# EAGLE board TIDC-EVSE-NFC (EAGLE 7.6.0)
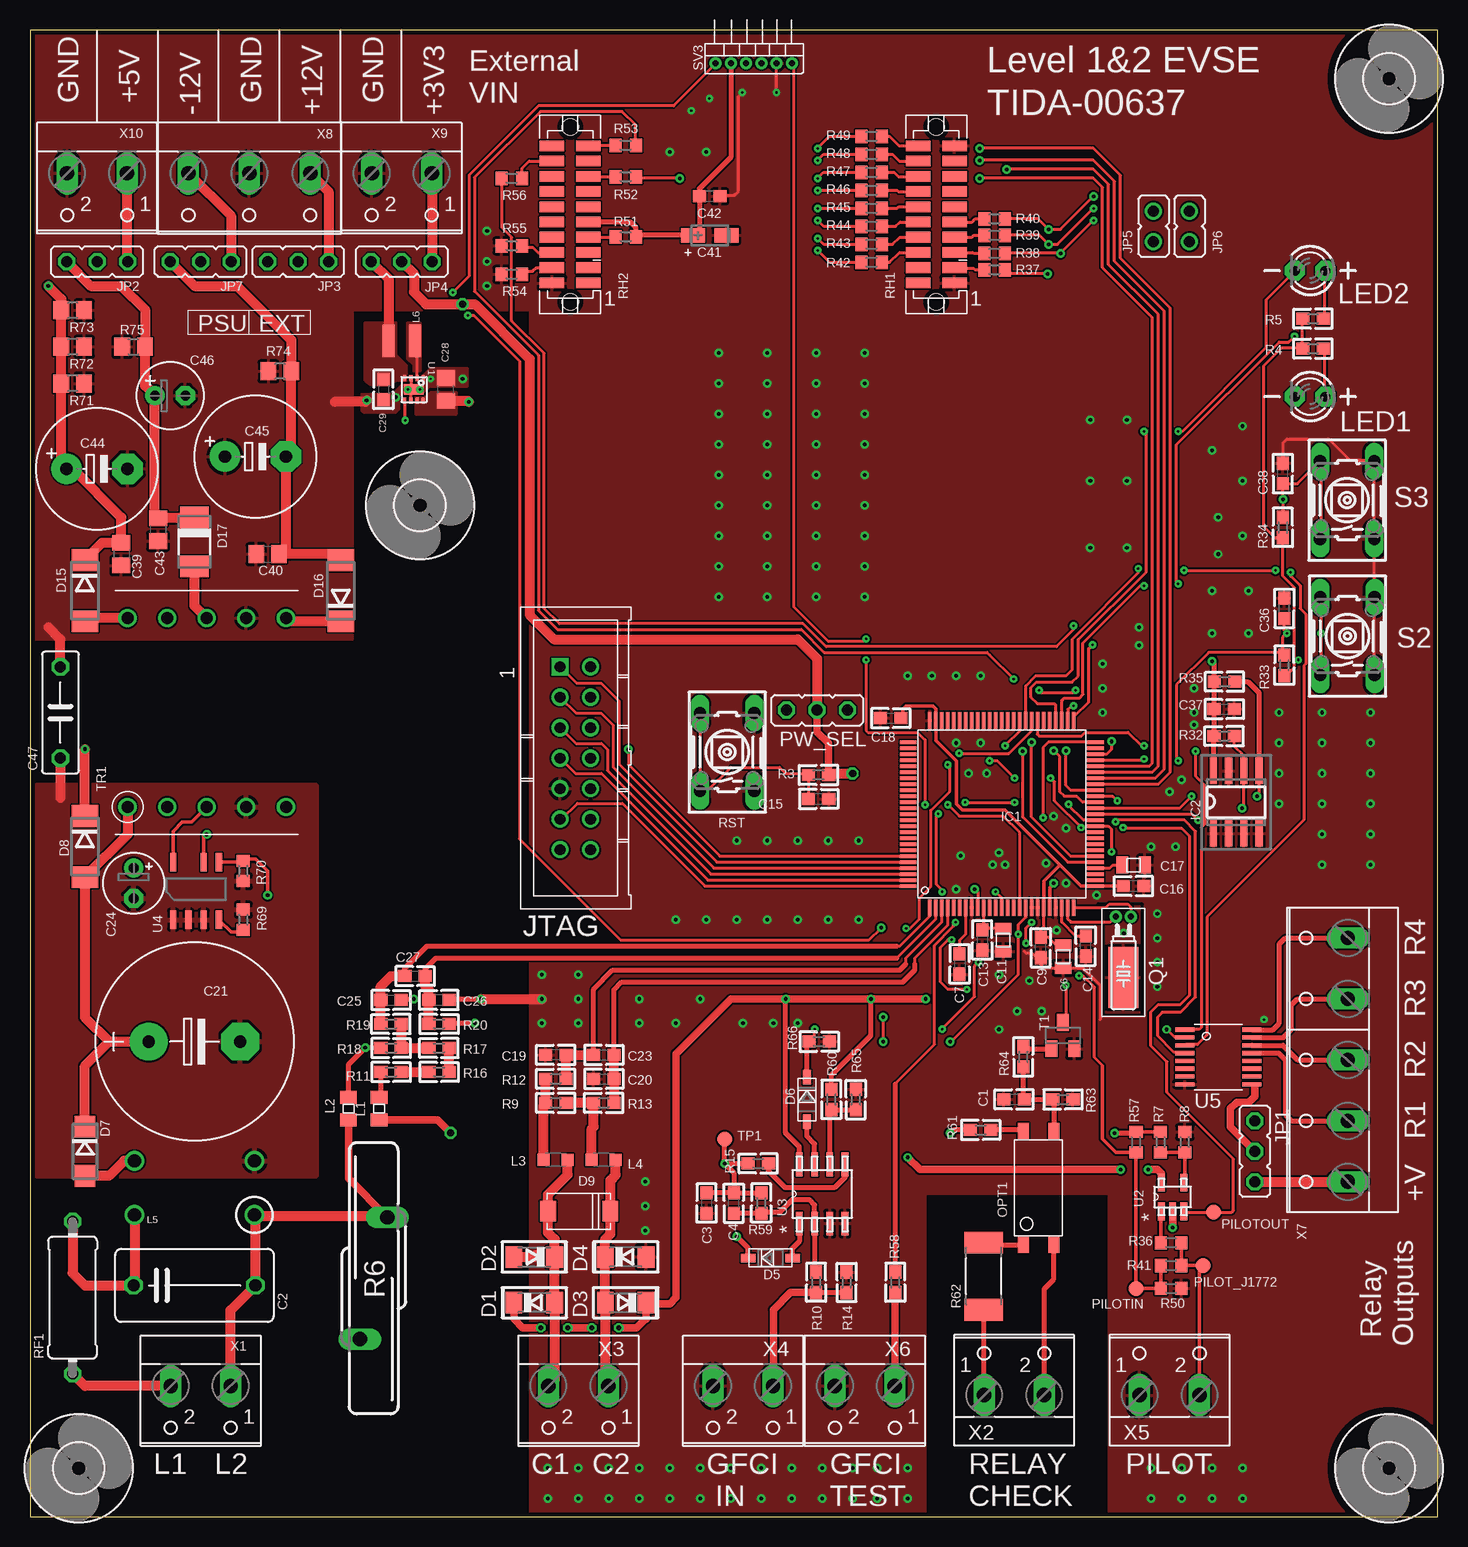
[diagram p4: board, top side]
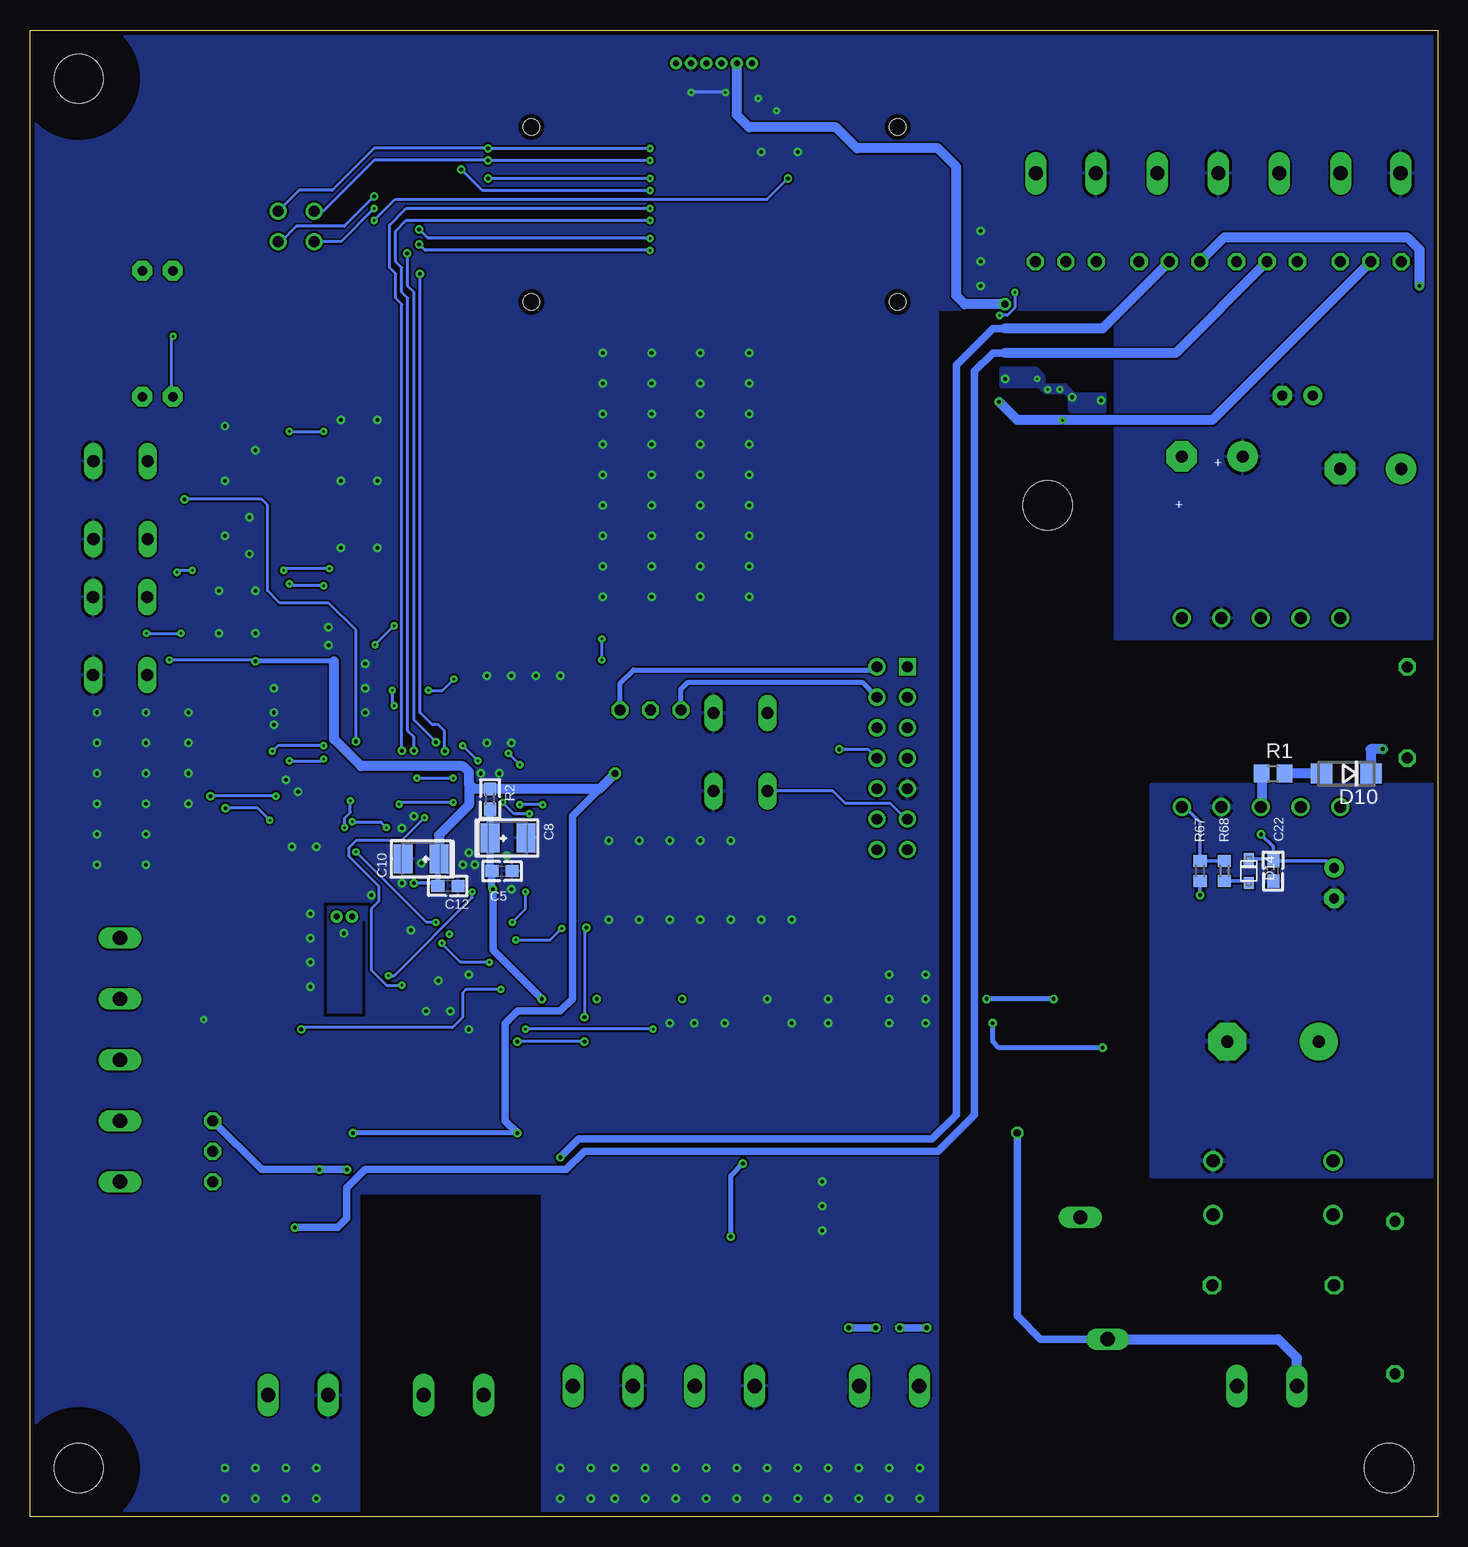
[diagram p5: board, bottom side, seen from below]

Size 117.35 x 123.95 mm. Coordinates in mm from the lower left corner, seen from the top.
Outline: 117.35,0 117.35,123.95 0,123.95 0,0 117.35,0
Copper layers (1*16): Top 0.0356mm / dielectric 1.5011mm / Bottom 0.0356mm
Design rules "typical_4pcb *": minimum track width 10mil, minimum drill 8mil, track to track 6mil, track to pad 6mil, pad to pad 6mil, via to via 6mil, smd to smd 6mil, copper to edge 15mil, drill to drill 8mil, minimum pad ring 10mil, minimum via ring 8mil, stop-mask expansion 4mil, vias tented up to drill 25mil, thermal gap 10mil
tRestrict: 4 lines
bRestrict: 4 lines

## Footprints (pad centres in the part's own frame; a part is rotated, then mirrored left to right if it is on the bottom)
C0603 = smd 1.1 x 1: 1 -0.85,0; 2 0.85,0
C102-064X133 = drill 1.016 octagon: 1 -5.08,0; 2 5.08,0
0805 = smd 1 x 1.4: 1 -0.94,0; 2 0.94,0
SMC_B = smd 1.6 x 2.4: + -1.5,0; - 1.5,0
E7,5-16 = drill 1.016 pad 3.15: + -3.81,0 | drill 1.016 pad 3.15 octagon: - 3.81,0
E2,5-5 = drill 0.813 pad 1.6: + -1.27,0 | drill 0.813 pad 1.6 octagon: - 1.27,0
C0805 = smd 1.3 x 1.5: 1 -0.95,0; 2 0.95,0
CT3216 = smd 2 x 1.2: + -1.4,0; - 1.4,0
E5-10,5 = drill 1.016 pad 2.54: + -2.54,0 | drill 1.016 pad 2.54 octagon: - 2.54,0
E2,5-6 = drill 0.813 pad 1.6: + -1.27,0 | drill 0.813 pad 1.6 octagon: - 1.27,0
C075-032X103 = drill 0.914 octagon: 1 -3.81,0; 2 3.81,0
SOD80C = smd 1.4 x 1.8: A -1.7,0; C 1.7,0
SOD-123 = smd 1.2 x 0.7: A 1.85,0; C -1.85,0
DO214AC = smd 1.8 x 1.7: A 2.05,0; C -2.05,0
DO214AA = smd 1.8 x 2.2: A 2.55,0; C -2.55,0
DO-214 = smd 1.3 x 1.7: 1 0,0; 2 5.2,0
SOD-323F = smd 1 x 0.8: A -1,0; C 1,0
DO-214AC = smd 1.8 x 2.4: A 2.025,0; C -2.025,0
4,1 = hole 4.1: 0,0
PZ100 = smd 1.4 x 0.3: 1 -7.8,6; 2 -7.8,5.5; 3 -7.8,5; 4 -7.8,4.5; 5 -7.8,4; 6 -7.8,3.5; 7 -7.8,3; 8 -7.8,2.5; 9 -7.8,2; 10 -7.8,1.5; 11 -7.8,1; 12 -7.8,0.5; 13 -7.8,0; 14 -7.8,-0.5; 15 -7.8,-1; 16 -7.8,-1.5; 17 -7.8,-2; 18 -7.8,-2.5; 19 -7.8,-3; 20 -7.8,-3.5; 21 -7.8,-4; 22 -7.8,-4.5; 23 -7.8,-5; 24 -7.8,-5.5; 25 -7.8,-6; 51 7.8,-6; 52 7.8,-5.5; 53 7.8,-5; 54 7.8,-4.5; 55 7.8,-4; 56 7.8,-3.5; 57 7.8,-3; 58 7.8,-2.5; 59 7.8,-2; 60 7.8,-1.5; 61 7.8,-1; 62 7.8,-0.5; 63 7.8,0; 64 7.8,0.5; 65 7.8,1; 66 7.8,1.5; 67 7.8,2; 68 7.8,2.5; 69 7.8,3; 70 7.8,3.5; 71 7.8,4; 72 7.8,4.5; 73 7.8,5; 74 7.8,5.5; 75 7.8,6 | smd 0.3 x 1.4: 26 -6,-7.8; 27 -5.5,-7.8; 28 -5,-7.8; 29 -4.5,-7.8; 30 -4,-7.8; 31 -3.5,-7.8; 32 -3,-7.8; 33 -2.5,-7.8; 34 -2,-7.8; 35 -1.5,-7.8; 36 -1,-7.8; 37 -0.5,-7.8; 38 0,-7.8; 39 0.5,-7.8; 40 1,-7.8; 41 1.5,-7.8; 42 2,-7.8; 43 2.5,-7.8; 44 3,-7.8; 45 3.5,-7.8; 46 4,-7.8; 47 4.5,-7.8; 48 5,-7.8; 49 5.5,-7.8; 50 6,-7.8; 76 6,7.8; 77 5.5,7.8; 78 5,7.8; 79 4.5,7.8; 80 4,7.8; 81 3.5,7.8; 82 3,7.8; 83 2.5,7.8; 84 2,7.8; 85 1.5,7.8; 86 1,7.8; 87 0.5,7.8; 88 0,7.8; 89 -0.5,7.8; 90 -1,7.8; 91 -1.5,7.8; 92 -2,7.8; 93 -2.5,7.8; 94 -3,7.8; 95 -3.5,7.8; 96 -4,7.8; 97 -4.5,7.8; 98 -5,7.8; 99 -5.5,7.8; 100 -6,7.8
SO-08 = smd 2.2 x 0.6: 1 -2.6,1.905; 2 -2.6,0.635; 3 -2.6,-0.635; 4 -2.6,-1.905; 5 2.6,-1.905; 6 2.6,-0.635; 7 2.6,0.635; 8 2.6,1.905
JP2 = drill 0.914 octagon: 1 -2.54,0; 2 0,0; 3 2.54,0
JP1 = drill 0.914: 1 0,-1.27; 2 0,1.27
MA07-2JTAG = drill 0.9 pad 1.422 square: 1 0,0 | drill 0.9 pad 1.422: 2 0,2.54; 3 2.54,0; 4 2.54,2.54; 5 5.08,0; 6 5.08,2.54; 7 7.62,0; 8 7.62,2.54; 9 10.16,0; 10 10.16,2.54; 11 12.7,0; 12 12.7,2.54; 13 15.24,0; 14 15.24,2.54
0805@1 = smd 1.092 x 1.397: 1 -0.94,0; 2 0.94,0
L2012C = smd 1 x 1: 1 -1,0; 2 1,0
744821110 = drill 1.1: 1 5,-2.25; 2 5,2.25; 3 -5,2.25; 4 -5,-2.25
SRN3015 = smd 2.7 x 1: V_1 0,1.1; V_2 0,-1.1
LED3MM = drill 0.8 pad 1.676 octagon: A -1.27,0; K 1.27,0
TCLT1600 = smd 1.3 x 0.9: 1 -4.75,1.27; 2 -4.75,-1.27; 3 4.75,-1.27; 4 4.75,1.27
B1,27 = smd 1.27 x 1.27: TP 0,0
TC26H-1 = drill 0.5 pad 1.016: 1 -0.635,0; 2 0.635,0 | smd 2.54 x 5.08: 3 0,5.08
R0805 = smd 1.3 x 1.5: 1 -0.95,0; 2 0.95,0
R0603 = smd 1.1 x 1: 1 -0.85,0; 2 0.85,0
S20K680-1 = drill 1.2 long: 1 -1.143,-5.08; 2 1.143,5.08
R0603' = smd 1 x 1.1: 1 -0.85,0; 2 0.85,0
R2512 = smd 1.8 x 3.2: 1 -2.8,0; 2 2.8,0
0411/12 = drill 0.914 octagon: 1 -6.35,0; 2 6.35,0
TFM-110-02-SM-D-A-K = smd 2.032 x 0.889: 1 -1.524,5.715; 2 1.524,5.715; 3 -1.524,4.445; 4 1.524,4.445; 5 -1.524,3.175; 6 1.524,3.175; 7 -1.524,1.905; 8 1.524,1.905; 9 -1.524,0.635; 10 1.524,0.635; 11 -1.524,-0.635; 12 1.524,-0.635; 13 -1.524,-1.905; 14 1.524,-1.905; 15 -1.524,-3.175; 16 1.524,-3.175; 17 -1.524,-4.445; 18 1.524,-4.445; 19 -1.524,-5.715; 20 1.524,-5.715 | hole 1.359: 0,7.303; 0,-7.303
B3F-10XX = drill 1.016 long: 1 -3.251,2.261; 2 3.251,2.261; 3 -3.251,-2.261; 4 3.251,-2.261
MA06-1-1.27 = drill 0.5 pad 0.9: 1 0,0; 2 1.27,0; 3 2.54,0; 4 3.81,0; 5 5.08,0; 6 6.35,0
SOT23 = smd 1 x 1.4: 1 -0.95,-1.1; 2 0.95,-1.1; 3 0,1.1
RLTI-1118 = drill 1: V_1 -7.874,6.604; V_2 -7.874,3.302; V_3 -7.874,0; V_4 -7.874,-3.302; V_5 -7.874,-6.604; V_6 7.874,-6.604; V_7 7.874,-3.302; V_8 7.874,0; V_9 7.874,3.302; V_10 7.874,6.604
DSG0008A = smd 0.508 x 0.254: 1 -0.94,0.762; 2 -0.94,0.254; 3 -0.94,-0.254; 4 -0.94,-0.762; 5 0.94,-0.762; 6 0.94,-0.254; 7 0.94,0.254; 8 0.94,0.762 | smd 0.889 x 1.6: 9 0,0
DBV5 = smd 1.473 x 0.559: 1 -1.194,0.94; 2 -1.194,0; 3 -1.194,-0.94; 4 1.194,-0.94; 5 1.194,0.94
M08A = smd 1.981 x 0.559: 1 -2.464,1.905; 2 -2.464,0.635; 3 -2.464,-0.635; 4 -2.464,-1.905; 5 2.464,-1.905; 6 2.464,-0.635; 7 2.464,0.635; 8 2.464,1.905
D0007A = smd 1.524 x 0.508: 1 0,3.81; 2 0,2.54; 3 0,1.27; 4 0,0; 5 4.801,0; 6 4.801,1.27; 8 4.801,3.81
TSSOP_16 = smd 1.6 x 0.35: V_1 -2.8,4.55; V_2 -2.8,3.9; V_3 -2.8,3.25; V_4 -2.8,2.6; V_5 -2.8,1.95; V_6 -2.8,1.3; V_7 -2.8,0.65; V_8 -2.8,0; V_9 2.8,0; V_10 2.8,0.65; V_11 2.8,1.3; V_12 2.8,1.95; V_13 2.8,2.6; V_14 2.8,3.25; V_15 2.8,3.9; V_16 2.8,4.55
W237-102 = drill 1.194 long: 1 -2.5,-1.27; 2 2.5,-1.27
W237-5P = drill 1.194 long: 1 -10.16,-0.635; 2 -5.08,-0.635; 3 0,-0.635; 4 5.08,-0.635; 5 10.16,-0.635
W237-133 = drill 1.194 long: 1 -5.08,-0.635; 2 0,-0.635; 3 5.08,-0.635

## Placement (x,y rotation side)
C1  47pF  [C0603]  82.04,34.8 180 top
C2  [C102-064X133]  13.72,19.3 0 top
C3  10u  [C0603]  56.39,26.16 270 top
C4  100n  [C0603]  58.67,26.16 90 top
C5  0.1uF  [C0603]  78,53.84 0 bottom
C6  4.7uF  [0805]  86.12,46.71 90 top
C7  0.1uF  [C0603]  77.5,46.09 270 top
C8  4.7uF  [SMC_B]  77.5,56.59 0 bottom
C9  4.7uF  [C0603]  84.25,47.46 90 top
C10  4.7uF  [SMC_B]  84.75,54.84 180 bottom
C11  4.7uF  [0805]  81.12,48.09 90 top
C12  0.1uF  [C0603]  82.5,52.59 180 bottom
C13  0.1uF  [C0603]  79.38,48.09 270 top
C14  0.47uF  [C0603]  88,47.59 90 top
C15  0.01uF  [C0603]  65.74,59.86 0 top
C16  0.47uF  [C0603]  92,52.59 180 top
C17  4.7uF  [0805]  92,54.34 180 top
C18  0.1uF  [C0603]  71.75,66.59 0 top
C19  47pF  [C0603]  43.83,38.52 180 top
C20  47pF  [C0603]  47.83,36.52 0 top
C21  [E7,5-16]  13.72,39.62 0 top
C22  .1u  [C0603]  13.72,53.85 90 bottom
C23  15nF  [C0603]  47.83,38.52 0 top
C24  22u  [E2,5-5]  8.64,52.83 270 top
C25  47pF  [C0603]  30.1,43.09 0 top
C26  47pF  [C0603]  34.1,43.09 180 top
C27  15nF  [C0603]  32.1,45.09 0 top
C28  4.7u  [C0805]  34.67,93.98 90 top
C29  10.0u  [C0603]  29.46,93.98 270 top
C36  0.1uF  [C0603]  104.56,75.74 90 top
C37  0.1uF  [C0603]  99.56,67.34 0 top
C38  0.1uF  [C0603]  104.44,86.98 90 top
C39  1u  [C0805]  7.62,80.26 270 top
C40  1u  [C0805]  19.81,80.26 0 top
C41  10uF  [CT3216]  56.66,106.83 0 top
C42  0.1uF  [C0603]  56.66,110.08 180 top
C43  1u  [C0805]  10.67,82.3 270 top
C44  680u  [E5-10,5]  5.59,87.38 0 top
C45  680u  [E5-10,5]  18.8,88.39 0 top
C46  220u  [E2,5-6]  11.68,93.47 0 top
C47  1000p  [C075-032X103]  2.54,67.06 90 top
D1  1N4148  [SOD80C]  42.04,17.87 180 top
D2  1N4148  [SOD80C]  42.04,21.68 0 top
D3  1N4148  [SOD80C]  49.66,17.87 0 top
D4  1N4148  [SOD80C]  49.66,21.68 180 top
D5  [SOD-123]  61.72,21.59 0 top
D6  [SOD-123]  64.77,34.8 270 top
D7  [DO214AC]  4.57,30.48 270 top
D8  [DO214AA]  4.57,55.88 270 top
D9  SMAJ5.0CA  [DO-214]  48.39,25.49 180 top
D10  [DO214AC]  7.62,61.98 180 bottom
D14  [SOD-323F]  15.75,53.85 90 bottom
D15  [DO214AA]  4.57,77.22 270 top
D16  [DO214AA]  25.91,77.22 90 top
D17  [DO-214AC]  13.72,81.28 270 top
H1  MOUNT-HOLE4.1  [4,1]  4.06,4.06 0 top
H2  MOUNT-HOLE4.1  [4,1]  113.28,4.06 0 top
H3  MOUNT-HOLE4.1  [4,1]  113.28,119.89 0 top
H4  MOUNT-HOLE4.1  [4,1]  32.51,84.33 0 top
IC1  F6733---PZ100  [PZ100]  81,58.59 90 top
IC2  24C02CSN  [SO-08]  100.56,59.59 90 top
JP1  [JP2]  102.11,30.48 270 top
JP2  [JP2]  5.59,104.65 180 top
JP3  [JP2]  22.35,104.65 180 top
JP4  [JP2]  30.99,104.65 180 top
JP5  [JP1]  93.66,107.58 0 top
JP6  [JP1]  96.66,107.58 0 top
JP7  [JP2]  14.22,104.65 180 top
JTAG  [MA07-2JTAG]  44.2,70.87 270 top
L1  EXCML20A  [0805@1]  29.09,34.04 90 top
L2  EXCML20A  [0805@1]  26.54,34.04 90 top
L3  BLM21BD121SN1D  [L2012C]  43.83,29.77 180 top
L4  BLM21BD121SN1D  [L2012C]  47.83,29.77 180 top
L5  744821110  [744821110]  13.72,27.43 0 top
L6  1u  [SRN3015]  30.99,98.04 90 top
LED1  [LED3MM]  106.71,93.38 180 top
LED2  [LED3MM]  106.71,103.88 180 top
OPT1  TCLT1600  [TCLT1600]  84.07,27.43 90 top
PILOT_J1772  TPB1,27  [B1,27]  97.79,20.95 270 top
PILOTIN  TPB1,27  [B1,27]  92.2,19.05 90 top
PILOTOUT  TPB1,27  [B1,27]  98.68,25.4 270 top
PW_SEL  [JP2]  65.62,67.26 180 top
Q1  32.768  [TC26H-1]  91.15,50.04 180 top
R1  33.2  [R0805]  13.72,61.98 0 bottom
R2  10 ohm  [R0603]  79,59.84 270 bottom
R3  47K  [R0603]  65.74,61.85 180 top
R4  100  [R0603]  106.96,97.38 180 top
R5  100  [R0603]  106.96,99.88 180 top
R6  S20K275  [S20K680-1]  28.65,19.89 180 top
R7  100k  [R0603']  94.23,31.24 90 top
R8  100k  [R0603']  96.27,31.24 270 top
R9  13R  [R0603]  43.83,34.52 180 top
R10  1K  [R0603]  65.53,19.56 270 top
R11  330K  [R0603]  30.1,37.09 0 top
R12  1K  [R0603]  43.83,36.52 180 top
R13  1K  [R0603]  47.83,34.52 180 top
R14  330  [R0603]  68.07,19.56 90 top
R15  150  [R0603]  60.71,29.46 180 top
R16  330K  [R0603]  34.1,37.09 0 top
R17  330K  [R0603]  34.1,39.09 180 top
R18  3K  [R0603]  30.1,39.09 0 top
R19  100  [R0603]  30.1,41.09 180 top
R20  1K  [R0603]  34.1,41.09 0 top
R32  10K  [R0603]  99.56,65.09 180 top
R33  100k  [R0603]  104.56,70.99 270 top
R34  100k  [R0603]  104.44,82.48 270 top
R35  10K  [R0603]  99.58,69.63 180 top
R36  910  [R0603']  95.12,22.86 0 top
R37  0  [R0603']  80.41,103.95 180 top
R38  0  [R0603']  80.41,105.33 180 top
R39  0  [R0603']  80.41,106.83 180 top
R40  0  [R0603']  80.41,108.2 180 top
R41  300k  [R0603']  95.12,20.95 0 top
R42  0  [R0603']  70.16,104.58 180 top
R43  0  [R0603']  70.16,106.08 180 top
R44  0  [R0603']  70.16,107.58 180 top
R45  0  [R0603']  70.16,109.08 180 top
R46  0  [R0603']  70.16,110.58 180 top
R47  0  [R0603']  70.16,112.08 180 top
R48  0  [R0603']  70.16,113.58 180 top
R49  0  [R0603']  70.16,115.08 180 top
R50  100k  [R0603']  95.12,19.05 180 top
R51  0  [R0603']  49.66,106.71 180 top
R52  0  [R0603']  49.66,111.71 180 top
R53  0  [R0603']  49.66,114.33 180 top
R54  0  [R0603']  40.16,103.58 180 top
R55  0  [R0603']  40.16,105.96 180 top
R56  0  [R0603']  40.16,111.58 180 top
R57  82k  [R0603']  92.2,31.24 90 top
R58  330  [R0603]  72.14,19.56 270 top
R59  100k  [R0603]  60.96,26.16 270 top
R60  150  [R0603]  66.8,34.8 270 top
R61  1K  [R0603]  79.25,32.26 0 top
R62  18k  [R2512]  79.5,20.07 90 top
R63  1K  [R0603]  86.11,34.8 0 top
R64  1K  [R0603]  82.8,38.35 90 top
R65  150  [R0603]  68.83,34.8 90 top
R66  10k  [R0603]  65.79,39.62 0 top
R67  33.2k  [R0603']  19.81,53.85 90 bottom
R68  10  [R0603']  17.78,53.85 90 bottom
R69  806  [R0603']  17.78,49.78 270 top
R70  15.0k  [R0603']  17.78,53.85 90 top
R71  2k  [R0805]  3.56,94.49 180 top
R72  2k  [R0805]  3.56,97.54 180 top
R73  2k  [R0805]  3.56,100.58 180 top
R74  2k  [R0805]  20.83,95.5 180 top
R75  511  [R0805]  8.64,97.54 0 top
RF1  [0411/12]  3.56,18.29 90 top
RH1  [TFM-110-02-SM-D-A-K]  75.55,108.58 180 top
RH2  [TFM-110-02-SM-D-A-K]  45.03,108.58 180 top
RST  [B3F-10XX]  58.12,63.76 90 top
S2  [B3F-10XX]  109.83,73.42 90 top
S3  [B3F-10XX]  109.8,84.76 90 top
SV3  [MA06-1-1.27]  57.16,121.19 0 top
T1  BC846  [SOT23]  86.11,40.13 0 top
TP1  TPB1,27  [B1,27]  57.91,31.5 90 top
TR1  RLTI-1118RLTI-1118  [RLTI-1118]  14.73,67.06 90 top
U1  TPS62063DSGR  [DSG0008A]  32,93.98 270 top
U2  OPA171  [DBV5]  95.25,26.67 90 top
U3  LM7321  [M08A]  66.04,26.92 90 top
U4  Value  [D0007A]  15.75,49.78 90 top
U5  TPL7407L  [TSSOP_16]  99.06,36.07 0 top
X1  [W237-102]  14.22,9.65 180 top
X2  [W237-102]  82.04,11.43 0 top
X3  [W237-102]  45.72,9.65 180 top
X4  [W237-102]  59.44,9.65 180 top
X5  [W237-102]  95,11.43 0 top
X6  [W237-102]  69.6,9.65 180 top
X7  [W237-5P]  109.22,38.1 90 top
X8  [W237-133]  18.29,111.38 180 top
X9  [W237-102]  30.99,110.74 180 top
X10  [W237-102]  5.59,110.74 180 top

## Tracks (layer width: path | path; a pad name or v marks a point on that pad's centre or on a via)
+3V3_S
  Top 0.813: JP4.3 29.89,103.21 L6.V_1
  pour Top (no thermals): 30.48,99.57 30.48,96.9 31.37,96.01 31.37,94.74 30.48,94.74 29.97,94.36 28.45,94.36 27.94,94.74 27.94,99.57
+5V  (via drill 0.2, 0.3)
  Top 0.254: v31.27,91.41 31.27,92.9 U1.5
  Top 0.813: v36.58,92.96 36.51,93.03 C28.1
  Bottom 0.254: v31.27,91.41 31.27,91.44
  Bottom 0.813: JP2.2 18.8,91.44 31.27,91.44 35.05,91.44 v36.58,92.96
  pour Top (no thermals): 35.56,93.73 33.4,93.73 33.02,93.34 32.13,93.34 32.13,91.95 35.56,91.95
+5V_S
  Top 0.813: D17.C 13.66,83.25 C43.1 10.41,83.5 C46.+ 9.59,94.3 R75.2 9.59,100.65 7.62,102.62 5.08,102.62 JP2.3
+12V  (via drill 0.3)
  Top 0.61: v73.15,29.97 74.17,28.96 v90.93,28.96 | v93.22,28.96 93.98,28.96 94.31,28.63 U2.5
  Bottom 0.61: v73.15,29.97 71.63,31.5 42.16,31.5 40.13,33.53 40.13,96.01 37.08,99.06 36.07,99.06 | JP1.1 98.04,28.96 v93.22,28.96 v90.93,28.96
  Bottom 0.813: JP3.2 27.94,99.06 36.07,99.06
+12V_S  (via drill 0.3)
  Top 0.813: D15.C 6.02,81.21 C39.1 7.62,83.31 3.56,87.38 C44.+ 2.61,87.82 R71.2 R72.2 R73.2 2.61,101.53 v1.52,102.62
  Bottom 0.813: JP3.3 17.78,106.68 2.54,106.68 1.52,105.66 v1.52,102.62
-12V  (via drill 0.3)
  Top 0.61: v95.25,24.13 U2.2
  Bottom 0.61: 36.07,97.03 37.08,97.03 38.61,95.5 38.61,33.53 41.66,30.48 71.12,30.48 72.64,28.96 89.41,28.96 90.93,27.43 90.93,24.89 91.69,24.13 v95.25,24.13
  Bottom 0.813: JP7.2 21.84,97.03 36.07,97.03
-12V_S
  Top 0.813: D16.A 25.41,80.26 C40.2 21.34,80.84 C45.- 21.78,88.83 R74.1 21.78,98.11 17.27,102.62 13.72,102.62 JP7.3
AVCC  (via drill 0.3, 0.38)
  Top 0.254: IC1.9 79,52.09 v78.75,52.34
  Top 0.406: R60.1 66.8,36.83 70.1,40.13 v70.1,43.18 | U3.8 64.14,30.86 62.99,32 v62.99,43.18
  Top 0.61: D1.C 40.34,16.51 41.08,15.77 v42.58,15.77 | v44.83,15.77 v46.83,15.77 | v49.08,15.77 50.58,15.77 51.36,16.54 D3.C | D3.C 51.36,16.49 | D3.C 51.44,17.78 53.34,17.78 53.85,18.29 53.85,38.61 58.42,43.18 v62.99,43.18 v70.1,43.18 v74.68,43.18
  Bottom 0.406: C5.1 79,54.24 | v78.75,52.34 78.85,52.44
  Bottom 0.61: R2.2 C8.+ 79,54.24 | 78.85,52.44 C5.1 | v78.75,52.34 | v42.58,15.77 v44.83,15.77 | v46.83,15.77 v49.08,15.77 | v74.68,43.18 78.75,47.25 v78.75,52.34
BT1  (via drill 0.3)
  Top 0.254: R34.1 104.46,83.5 v104.46,84.84 104.46,86.04 C38.1 105.66,86.13 S3.2 107.63,87.95 107.63,81.6 S3.1 | IC1.48 89.75,63.59 90.17,64.01 v90.17,64.64
  Bottom 0.254: v90.17,64.64 90.17,73.91 92.46,76.2 96.52,76.2 97.54,77.22 97.54,84.33 98.04,84.84 v104.46,84.84
BT2  (via drill 0.2)
  Top 0.254: 104.46,74.61 C36.1 | S2.2 107.63,76.52 v107.63,73.66 107.63,70.48 S2.1 | 104.78,74.61 C36.1 | v95.73,63.02 95.57,63.18 95.57,69.37 98.27,72.07 104.46,72.07 | 104.46,72.07 R33.1 | IC1.47 92.77,63.09 v92.87,63.18 | 104.46,72.07 104.46,73.34 v104.78,73.66 104.56,73.87 C36.1
  Top 0.406: C36.1 104.65,74.68
  Bottom 0.254: v107.63,73.66 v104.78,73.66 | v92.87,63.18 93.03,63.02 v95.73,63.02
CUR1+
  Top 0.813: L3.1 44.83,28.52 43.19,26.87 D9.2 43.19,23.7 43.74,23.15 D2.C D1.A 43.74,11.44 X3.2
CUR1-
  Top 0.813: L4.1 48.83,28.52 48.39,28.07 D9.1 48.39,23.58 47.96,23.15 D4.C D3.A 47.96,11.19 X3.1
DVCC  (via drill 0.2, 0.3, 0.6)
  Top 0.254: 98.65,62.1 IC2.8 | 106.05,97.47 106.05,99.69 R5.2 | 105.41,71.44 105.41,70.8 104.78,70.17 R33.2 | 105.41,71.44 105.41,77.47 104.46,78.42 104.46,81.6 R34.2 104.14,81.6 103.82,81.6 102.87,82.55 102.87,95.99 104.35,97.47 106.05,97.47 | 106.05,97.47 R4.2 | v105.73,71.44 105.41,71.44
  Top 0.305: R7.2 R57.2 | IC1.21 85,52.49 v85.34,52.83
  Top 0.406: IC2.8 98.65,65.03 R32.2 C37.1 98.71,69.6 | 98.71,69.6 R35.2 | 98.71,69.6 98.71,71.19 v98.56,71.34 | SV3.2 58.43,113.35 55.81,110.73 C42.2 55.81,107.38 C41.+ 50.63,106.83 R51.1 50.51,107.48 50.05,107.94 RH2.9 | R61.1 76.96,32.26 v76.71,32 | v90.42,32 92.11,32 R57.2
  Top 0.61: PW_SEL.2 65.62,65.44 66.55,64.52 66.55,61.89 R3.1
  Top 0.813: JP4.2 32,103.63 32,102.11 33.02,101.09 v36.07,101.09 37.08,101.09 41.66,96.52 41.66,75.18 43.69,73.15 64.01,73.15 65.62,71.54 PW_SEL.2 | R3.1 66.71,61.98 v68.58,61.98
  Bottom 0.254: v98.56,71.34 | v105.73,71.44 98.74,71.44 v98.56,71.34
  Bottom 0.305: C12.2 83.59,52.83 v85.34,52.83
  Bottom 0.406: 83.35,54.8 C12.2 | 92,71.34 v98.56,71.34 | v76.71,32 v90.42,32
  Bottom 0.61: v76.71,32 77.72,33.02 77.72,41.15 76.71,42.16 73.15,42.16 72.14,43.18 72.14,58.42 v68.58,61.98
  Bottom 0.813: 92,71.34 92,64.84 89.75,62.59 81.25,62.59 80.75,62.09 80.75,61.09 | 83.35,54.8 C10.+ 83.25,56.84 80.75,59.34 80.75,61.09 | 80.75,61.09 80.35,60.69 R2.1 69.87,60.69 v68.58,61.98 | v36.07,101.09 39.41,101.09 40.13,101.81 40.13,112.55 41.66,114.08 48.41,114.08 50.16,115.83 57.41,115.83 58.43,116.85 SV3.2
GFCI+
  Top 0.406: R10.2 R14.1
  Top 0.61: R10.2 63.41,18.71 61.98,17.27 61.98,10.96 X4.1
GFCI_FAULT  (via drill 0.2)
  Top 0.254: v90.17,55.44 90.17,57.3 89.88,57.59 IC1.36 | v83.5,49.56 83.03,49.09 v83.03,47.82 | v79.06,46.23 78.74,45.91 78.74,43.37 v76.04,40.67 | v65.41,40.67 65.41,39.56 65.09,39.56 R66.1
  Top 0.406: D6.C 64.77,39.46 R66.1
  Bottom 0.254: v90.17,55.44 84.3,49.56 v83.5,49.56 | v83.03,47.82 81.44,46.23 v79.06,46.23 | v65.41,40.67 v76.04,40.67
GFCI_TEST  (via drill 0.2)
  Top 0.254: v86.58,59.4 86.58,59.32 87.82,58.09 IC1.37 | v77.95,59.56 v82.07,59.56 | v75.72,58.61 75.56,58.45 75.56,52.74 76.04,52.26 v76.04,52.1 | v77.15,49.56 76.99,49.4 76.99,49.24 75.41,47.66 75.41,39.4 72.23,36.23 72.14,36.07
  Top 0.406: R58.1 72.14,36.07
  Bottom 0.254: v86.58,59.4 86.42,59.56 v82.07,59.56 | v77.95,59.56 76.99,58.61 v75.72,58.61 | v76.04,52.1 76.04,50.67 v77.15,49.56
GND  (via drill 0.15, 0.2, 0.3)
  Top 0.254: U1.3 31.75,94.23 v31.5,93.98 31.75,93.73 U1.6 | 89.22,41.47 89.22,44.32 87.79,45.75 86.36,45.75 86.2,45.59 86.04,45.59 85.88,45.75 84.3,45.75 84.3,46.23 83.5,47.02 83.03,47.02 82.87,47.18 | 81.44,47.18 81.28,47.34 80.8,47.34 80.8,47.18 | v62.23,118.75 62.23,120.97 SV3.5 | v59.37,118.75 59.05,118.43 59.05,110.49 58.74,110.17 57.78,110.17 C42.1 | S2.3 112.08,70.48 112.08,76.52 S2.4 112.08,76.83 112.08,81.28 S3.3 112.08,81.6 112.08,87.95 S3.4 111.92,88.11 110.01,88.11 108.27,89.85 104.78,89.85 104.46,89.53 104.46,87.85 C38.2 104.3,87.95 104.14,88.11
  Top 0.406: 34.95,43.18 v37.59,43.18 | C25.2 30.95,43.18 v32,43.18
  Top 0.813: C47.2 2.54,73.15 1.52,74.17 | v28.07,93.09 27.94,92.96 25.4,92.96 | C26.1 34.95,43.18 | v37.59,43.18 v42.67,43.18 | D2.A 42,21.68 42.16,21.84
  Bottom 0.254: v59.37,118.75 v62.23,118.75
  Bottom 0.406: v32,43.18 v37.59,43.18
  other vias: 33.4,94.87 30.48,93.34 32.51,93.98 36.07,94.87 102.87,41.47 80.26,54.36 80.77,55.37 85.34,58.42 88.9,51.82 77.22,52.32 77.6,55.12 78.23,61.98 79.76,61.98 79.25,64.52 77.22,64.52 95,60.45 96.01,61.47 97.03,66.04 97.03,67.06 97.03,69.09 81.28,54.36 86.36,57.4 91.19,48.64 85.6,48.9 73.15,70.1 75.18,70.1 77.22,70.1 79.25,70.1 107.7,67.06 111.76,67.06 111.76,64.52 107.7,64.52 107.7,61.98 111.76,61.98 101.6,77.22 101.6,73.66 98.55,73.66 98.55,77.22 99.06,80.26 99.06,83.31 101.09,81.79 101.09,86.36 98.55,88.9 101.09,90.93 88.39,80.77 88.39,86.36 91.44,86.36 91.44,80.77 88.39,91.44 91.44,91.44 56.64,118.24 55.12,117.22 53.34,113.79 56.39,113.79 51.31,23.88 51.31,25.91 51.31,27.94 59.44,41.15 61.98,41.15 64.01,41.15 64.01,49.78 66.55,49.78 69.09,49.78 61.47,49.78 58.93,49.78 56.39,49.78 53.85,49.78 53.85,41.15 50.8,41.15 50.8,43.18 55.88,43.18 42.67,45.21 45.72,45.21 45.72,41.15 42.67,41.15 45.72,43.18 43.18,1.52 45.72,1.52 48.26,1.52 50.8,1.52 53.34,1.52 55.88,1.52 58.42,1.52 60.96,1.52 63.5,1.52 66.04,1.52 68.58,1.52 70.61,1.52 73.15,1.52 43.18,4.06 45.72,4.06 48.26,4.06 50.8,4.06 53.34,4.06 55.88,4.06 58.42,4.06 60.96,4.06 63.5,4.06 66.04,4.06 68.58,4.06 70.61,4.06 73.15,4.06 93.47,1.52 96.01,1.52 98.55,1.52 101.09,1.52 93.47,4.06 96.01,4.06 98.55,4.06 101.09,4.06 107.7,59.44 111.76,59.44 111.76,56.9 107.7,56.9 107.7,54.36 111.76,54.36 57.4,97.03 61.47,97.03 61.47,94.49 57.4,94.49 57.4,91.95 61.47,91.95 57.4,89.41 61.47,89.41 61.47,86.87 57.4,86.87 65.53,97.03 69.6,97.03 69.6,94.49 65.53,94.49 65.53,91.95 69.6,91.95 65.53,89.41 69.6,89.41 69.6,86.87 65.53,86.87 61.47,84.33 57.4,84.33 57.4,81.79 61.47,81.79 57.4,79.25 61.47,79.25 61.47,76.71 57.4,76.71 69.6,84.33 65.53,84.33 65.53,81.79 69.6,81.79 65.53,79.25 69.6,79.25 69.6,76.71 65.53,76.71 104.14,67.06 104.14,64.52 104.14,61.98 104.14,59.44 89.41,67.06 89.41,69.09 89.41,71.12 92.46,72.64 92.46,74.17 86.36,52.83 83.31,44.7 80.77,45.21 84.33,42.16 82.3,42.16 80.77,40.64 64.01,56.39 66.55,56.39 69.09,56.39 61.47,56.39 58.93,56.39 93.98,50.29 93.98,48.26 93.98,46.23 93.98,44.2 84.71,54.48 95.5,55.88 93.47,55.88 38.1,104.65 38.1,107.19 38.1,102.62
  pour Top: 41.66,-3.05 74.68,-3.05 74.68,26.92 89.92,26.92 89.92,-3.05 119.89,-3.05 119.89,127.51 -1.02,127.51 -1.02,73.15 26.92,73.15 26.92,100.58 41.66,100.58
  pour Top: 86.32,52.32 91.15,52.32 91.65,51.56 92.67,51.31 92.67,41.91 89.62,41.91 89.62,49.28 87.08,49.28 86.07,50.29 86.07,52.07
  pour Top (no thermals): 36.45,94.23 33.27,94.23 32.77,93.73 31.11,93.73 30.73,93.34 30.73,92.33 30.48,92.08 27.81,92.08 27.69,92.2 27.69,93.6 30.23,93.6 30.99,94.36 32.77,94.36 32.77,95.12 33.4,95.76 36.45,95.76
  pour Bottom (no thermals): 36.45,94.23 33.27,94.23 32.77,93.73 31.11,93.73 30.73,93.34 30.73,92.33 30.48,92.08 27.81,92.08 27.69,92.2 27.69,93.6 30.23,93.6 30.99,94.36 32.77,94.36 32.77,95.12 33.4,95.76 36.45,95.76
  pour Bottom: 41.66,-2.03 74.68,-2.03 74.68,26.92 89.92,26.92 89.92,-2.03 120.9,-2.03 120.9,128.52 -2.03,128.52 -2.03,73.15 26.92,73.15 26.92,100.58 41.66,100.58
I+
  Top 0.254: IC1.3 76,49.59 73,46.59 73,46.09
  Top 0.406: C23.1 46.98,43.99 48.58,45.59 72.5,45.59 73,46.09
  Top 0.813: R12.1 C19.1 | C19.1 | C19.1 C23.1
I-
  Top 0.254: IC1.4 76.5,49.34 73.75,46.59 73.75,46.09
  Top 0.406: 73.75,46.09 73.75,45.59 72.75,44.59 49.33,44.59 48.68,43.94 C23.2
  Top 0.813: C20.2 R13.1 | C20.2 | C20.2 C23.2 | C23.2
JTAG_EXT
  Bottom 0.406: PW_SEL.3 63.08,69 62.48,69.6 48.01,69.6 JTAG.4
JTAG_INT
  Bottom 0.406: PW_SEL.1 68.16,69.51 67.06,70.61 46.99,70.61 JTAG.2
LCDCAP
  Top 0.254: IC1.29 90,54.09 90.25,54.34 C17.2 | C17.2
LED1  (via drill 0.2)
  Top 0.254: v105.41,98.42 104.93,97.95 104.14,97.95 95.57,89.38 95.57,77.95 v95.73,77.79 | v92.87,77.63 92.55,77.63 87.79,72.87 87.79,68.58 87.47,68.26 86.2,68.26 86,68.06 IC1.53
  Bottom 0.254: v105.41,98.42 105.57,98.42 105.57,93.52 LED1.K | v95.73,77.79 95.57,77.63 v92.87,77.63
LED2  (via drill 0.2)
  Top 0.254: v92.87,90.49 93.03,90.33 93.03,78.74 87.38,73.15 87.38,70.1 86.87,69.6 83.88,69.6 83.44,69.15 83.44,68.33 83.98,67.79 85.41,67.79 85.5,67.69 IC1.54 | v95.73,90.49 96.04,90.49 103.03,97.47 103.03,101.44 105.41,103.82 LED2.K
  Bottom 0.254: v95.73,90.49 v92.87,90.49
LINE-VA
  Top 0.406: R11.1 29.25,35.13 L1.2
N$1
  Top 0.254: U1.2 32.26,97.87 L6.V_2
  pour Top (no thermals): 31.5,99.57 32.51,99.57 32.51,95.5 32,95.5 32,96.01 31.5,96.52
N$2
  Top 0.305: U2.4 96.27,27.94 R8.2 R7.1
N$3
  Top 0.813: X8.1 24.89,110.49 JP3.1
N$4
  Top 0.305: U2.1 94.27,25.44 R36.1
N$5
  Top 0.406: C4.1 R59.2 61.05,25.4 62.48,25.4 63.5,26.42 65.02,26.42 65.41,26.04 U3.2 65.41,20.54 R10.1
N$6
  Top 0.61: X6.1 72.1,18.67 R58.2
N$7
  Top 0.813: X8.3 16.76,108.46 JP7.1
N$8
  Top 0.406: U3.1 64.14,22.99 63.5,22.35 63.5,21.66 D5.A
N$9
  Top 0.406: R62.2 79.69,22.68 OPT1.1
N$10
  Top 0.406: R64.1 82.8,34.89 C1.1 R63.1 85.34,34.71 OPT1.3
N$11  (via drill 0.3)
  Top 0.406: C4.2 C3.1 | C4.2 R59.1 | D5.C 59.87,22.42 v58.93,23.37 | v57.91,29.46 R15.2 | v57.91,29.46 58.67,28.7 C4.2 | v57.91,29.46 TP1.TP
  Bottom 0.406: v58.93,23.37 58.93,28.45 v57.91,29.46
N$12
  Top 0.813: X9.1 33.53,113.5 JP4.1
N$13
  Top 0.813: JP2.1 8.09,104.69 X10.1
N$14
  Top 0.406: OPT1.4 82.73,32.26 R61.2
N$15
  Top 0.813: RF1.2 3.56,20.32 4.57,19.3 C2.1 8.72,19.38 L5.4
N$16
  Top 0.406: R15.1 61.56,28.87 62.99,27.43 67.06,27.43 67.94,28.32 U3.5
N$17
  Top 0.406: U3.6 66.67,33.82 R60.2 R65.1
N$18
  Top 0.813: L5.3 7.84,29.68 6.6,28.45 4.59,28.45 D7.A
N$19
  Top 0.406: U3.7 65.41,31.11 64.77,31.75 D6.A
N$20
  Top 0.813: D7.C 4.57,37.59 6.6,39.62 | 6.6,39.62 C21.+ | 6.6,39.62 4.57,41.66 D8.A 8.13,56.89 TR1.V_1
N$21
  Top 0.406: R64.2 82.98,39.03 T1.1
N$22  (via drill 0.3)
  Top 0.813: D8.C v4.57,64.01
  Bottom 0.813: v4.57,64.01 5.59,64.01 5.59,61.99 D10.C
N$23  (via drill 0.3)
  Top 0.406: R18.1 27.97,39.09 v27.94,39.12 26.54,37.72 L2.2 | v37.08,41.15 35.01,41.15 R20.2
  Bottom 0.406: v27.94,39.12 36.58,39.12 37.08,39.62 v37.08,41.15
N$24
  Bottom 0.813: D10.A R1.2
N$25
  Top 0.813: R16.2 R17.1
N$27
  Top 0.813: L4.2 46.83,32.37 46.98,32.52 R13.2 R9.1
N$30
  Top 0.305: U4.8 11.94,57.15 12.7,57.91 13.46,57.91 TR1.V_3
  Bottom 0.813: R1.1 14.67,59.25 TR1.V_3
N$32
  Top 0.813: R17.2 R18.2 R19.1
N$35
  Top 0.254: R37.2 78.78,103.95 78.66,104.08 77.13,104.08 RH1.3
N$36
  Bottom 0.305: TR1.V_5 21.08,59.18 19.81,57.91 R67.2 R68.2
N$37
  Bottom 0.305: R68.1 15.9,53 D14.A
N$38  (via drill 0.3)
  Top 0.305: U4.6 14.48,56.9 v14.73,56.9
  Bottom 0.305: v14.73,56.9 13.72,55.88 C22.2 | D14.C 13.87,54.85 C22.2 | C22.2 9.23,54.7 C24.+
N$39
  Top 0.813: R11.2 R16.1
N$40
  Top 0.813: TR1.V_6 21.6,74.67 D16.C
N$41
  Top 0.813: TR1.V_10 4.84,74.93 D15.A
N$42
  Top 0.813: L3.2 42.83,34.37 R9.2 R12.2 | R12.2
N$43
  Top 0.813: TR1.V_8 13.72,75.95 D17.A
N$45
  Top 0.254: RH1.5 78.58,105.41 78.66,105.33 R38.2
N$48  (via drill 0.3)
  Top 0.305: U4.5 17.67,54.59 R70.2 17.95,54.86 18.8,54.86 19.81,53.85 v19.81,51.82
  Bottom 0.305: R67.1 v19.81,51.82
N$49
  Top 0.305: U4.4 16.76,48.77 17.61,48.77 R69.2
N$50
  Top 0.254: RH2.7 48.78,106.67 R51.2
N$51
  Top 0.254: RH2.4 42.22,104.14 41.91,103.83 41.26,103.83 R54.1
N$52
  Top 0.254: R52.2 46.6,111.7 RH2.15
N$53
  Top 0.254: RH2.6 42.34,105.41 41.91,105.83 41.13,105.83 R55.1
N$55
  Top 0.254: R44.1 72.16,107.58 72.53,107.94 RH1.10
N$56
  Top 0.254: R45.1 72.28,109.08 72.41,109.2 74.02,109.2 RH1.12
N$57
  Top 0.254: R46.1 72.28,110.58 72.41,110.45 74,110.45 RH1.14
N$59
  Top 0.254: R47.1 72.03,112.08 72.41,111.7 73.98,111.7 RH1.16
N$60
  Top 0.254: R48.1 71.91,113.58 72.47,113.03 RH1.18
N$61
  Top 0.254: R49.1 71.66,115.08 72.44,114.3 RH1.20
N$81
  Top 0.254: R53.2 46.59,114.33 RH2.19
N$83
  Top 0.254: RH2.18 41.6,113.03 41.01,112.43 R56.1
N$85
  Top 0.254: RH1.7 78.5,106.67 78.66,106.83 R39.2
N$86
  Top 0.254: R40.2 78.78,108.2 78.53,107.94 RH1.9
N$87
  Top 0.254: R43.1 71.91,106.08 72.5,106.67 RH1.8
N$88
  Top 0.254: 73.98,105.45 RH1.6 72.48,105.41 71.66,104.58 R42.1
N$104
  Top 0.254: 107.81,93.55 LED1.A 107.95,93.66 107.95,97.16 R4.1
N$105
  Top 0.254: LED2.A 107.95,103.82 107.95,100.01 R5.1
PE
  Top 0.813: C47.1 2.54,59.94
  pour Bottom: -0.51,28.45 -0.51,60.96 23.88,60.96 23.88,28.45
  pour Top: 0.51,60.96 0.51,28.45 23.88,28.45 23.88,60.96
PILOT_J1772
  Top 0.305: R36.2 R41.2 PILOT_J1772.TP 97.5,20.66 X5.2
PILOTIN  (via drill 0.2)
  Top 0.254: v80.49,52.1 80.96,51.63 80.96,50.83 IC1.13 | v87.47,45.12 87.79,45.12 88.74,44.16 88.74,38.29 89.38,37.66 89.41,37.59
  Top 0.305: R41.1 R50.2 PILOTIN.TP R57.1 90.51,30.39 89.41,31.5 89.41,37.59
  Bottom 0.254: v87.47,45.12 87,45.12 80.49,51.63 v80.49,52.1
PILOTOUT  (via drill 0.2)
  Top 0.254: U2.3 96.2,25.4 PILOTOUT.TP 100.17,25.4 100.33,25.56 100.33,29.84 94.77,35.4 94.77,37.94 93.41,39.31 93.41,42.07 94.04,42.7 95.89,42.7 96.68,43.5 96.68,56.74 96.01,57.4 91.19,57.4 v91.12,57.47 | IC1.41 90.25,60.09 v90.65,59.69
  Bottom 0.254: v90.65,59.69 90.65,58.74 91.12,58.26 v91.12,57.47
R_SUP_J
  Top 0.813: JP1.3 X7.1
RELAY1  (via drill 0.2)
  Top 0.254: v97.16,63.82 97.16,61.75 97.95,60.96 97.95,57.78 97.63,57.47 97.63,40.8 97.47,40.64 96.36,40.64 U5.V_1 | v92.87,64.29 92.65,64.29 91.53,65.41 87.95,65.41 87.63,65.09 84.14,65.09 83.98,65.25 83.98,66.36 IC1.57
  Bottom 0.254: v92.87,64.29 96.68,64.29 v97.16,63.82
RELAY1_O
  Top 0.406: U5.V_16 103.61,40.62 104.14,41.15 104.14,47.75 104.65,48.26 X7.5
RELAY2  (via drill 0.2, 0.3)
  Top 0.254: v77.47,63.66 81.6,63.66 83.5,65.56 83.5,66.36 IC1.58 | v76.52,62.71 76.68,62.55 76.68,60.48 75.09,58.9 75.09,52.55 74.14,51.59 74.14,49.85 73.34,49.05 v73.03,49.05 | v76.83,48.1 76.52,48.1 75.88,47.47 75.88,44.61 76.52,43.97 v78.11,43.97 | U5.V_2 96.2,40.01 95.41,40.01 94.77,40.64 v94.74,40.64
  Bottom 0.254: v76.52,62.71 v77.47,63.66 | v73.03,49.05 73.98,48.1 v76.83,48.1 | v94.74,40.64 94.58,40.8 82.14,40.8 81.28,41.66 81.28,43.69 80.99,43.97 v78.11,43.97
RELAY2_O
  Top 0.406: U5.V_15 104.48,39.97 105.16,40.64 105.16,42.67 105.66,43.18 X7.4
RELAY3  (via drill 0.2)
  Top 0.254: v105.09,78.74 105.09,78.42 105.89,77.63 105.89,75.72 106.36,75.25 106.36,71.12 106.2,70.96 106.2,58.1 98.11,50.01 98.11,40.16 97.31,39.37 96.36,39.37 U5.V_3 | v96.2,78.9 v103.82,78.9 | v92.39,79.06 92.39,78.74 86.87,73.15 86.87,70.61 86.36,70.1 83.82,70.1 83,69.28 IC1.59
  Bottom 0.254: v105.09,78.74 104.93,78.9 v103.82,78.9 | v96.2,78.9 96.04,79.06 v92.39,79.06
RELAY3_O
  Top 0.406: U5.V_14 104.45,39.32 105.66,38.1 X7.3
RELAY4  (via drill 0.2)
  Top 0.254: v80.01,63.02 80.64,63.02 v82.07,61.59 | v85.09,61.59 85.41,61.28 85.41,59.69 v87.63,57.47 87.47,57.63 | v90.49,57.94 90.65,58.1 96.21,58.1 97.16,57.16 97.16,43.34 95.89,42.07 94.39,42.07 93.98,41.66 93.98,40.13 95.37,38.73 96.2,38.73 U5.V_4 | IC1.60 82.5,65.51 v81.28,64.29
  Bottom 0.254: v80.01,63.02 v81.28,64.29 | v85.09,61.59 v82.07,61.59 | v87.63,57.47 88.11,57.94 v90.49,57.94
RELAY4_O
  Top 0.406: U5.V_13 104.08,38.67 104.65,38.1 104.65,33.53 105.16,33.02 X7.2
RELAY_SUP
  Top 0.305: 102.11,35.82 U5.V_9
  Top 0.61: JP1.2 100.08,32.51 100.08,34.04 100.58,34.54 101.6,34.54 102.11,35.05 102.11,35.82
RESET
  Top 0.254: JTAG.11 44.32,58.17 45.63,59.47 49.38,59.47 56.27,52.59 IC1.100 | RST.2 RST.1 56.44,60.51 58.42,62.48 62.48,62.48 62.99,61.98 64.77,61.98 R3.2 C15.1
  Bottom 0.254: JTAG.11 44.32,58.17 45.63,59.47 49.38,59.47 50.41,60.51 RST.1 | 55.87,67.51 RST.2
RF_CCA  (via drill 0.2, 0.3)
  Top 0.254: R44.2 66.16,107.58 v65.66,108.08 | v85.34,63.88 85.85,63.37 85.85,60.45 86.22,60.09 87.23,60.09 87.73,59.59 IC1.40
  Bottom 0.254: v65.66,108.08 85.98,108.08 86.87,107.19 86.87,104.65 86.36,104.14 86.36,102.11 85.85,101.6 85.85,65.53 85.34,65.02 v85.34,63.88
RF_CLK  (via drill 0.2, 0.3)
  Top 0.254: IC1.46 93.31,62.59 93.56,62.84 93.56,99.99 89.41,104.14 89.41,110.83 88.66,111.58 v79.16,111.58 | R47.2 66.16,112.08 v65.66,111.58
  Bottom 0.254: v79.16,111.58 v65.66,111.58
RF_CS  (via drill 0.2, 0.3)
  Top 0.254: IC1.45 93.56,62.09 94.06,62.59 94.06,100.25 89.91,104.4 89.91,111.08 88.66,112.33 v81.41,112.33 | v65.66,110.58 R46.2 | v65.66,110.58
  Bottom 0.254: v81.41,112.33 79.66,110.58 v65.66,110.58
RF_FIFO  (via drill 0.2, 0.3)
  Top 0.254: R42.2 66.66,104.58 v65.66,105.58 | v88.66,109.08 85.66,106.08 v84.91,106.08 84.16,106.83 R39.1
  Bottom 0.254: v65.66,105.58 84.41,105.58 v84.91,106.08 | JP5.1 91.43,106.31 v88.66,109.08
RF_FIFOP  (via drill 0.2, 0.3)
  Top 0.254: R43.2 66.16,106.08 v65.66,106.58 | v88.66,110.08 85.91,107.33 v84.91,107.33 84.03,108.2 R40.1
  Bottom 0.254: v65.66,106.58 84.16,106.58 v84.91,107.33 | JP6.1 96.43,106.31 95.16,107.58 91.16,107.58 v88.66,110.08
RF_GPIO1  (via drill 0.2)
  Top 0.254: v87,67.63 86.84,67.63 86.52,67.31 86.52,66.52 IC1.52 | v87.15,68.9 87,68.74 84.3,68.74 v84.14,68.9 | R53.1 50.48,114.46 50.48,116.05 49.37,117.16 42.55,117.16 37.05,111.66 37.05,102.17 42.39,96.84 42.39,75.56 43.97,73.98 64.29,73.98 66.2,72.07 79.79,72.07 79.99,71.87 v82.01,69.85
  Bottom 0.254: v87,67.63 87.15,67.79 v87.15,68.9 | v84.14,68.9 82.96,68.9 v82.01,69.85
RF_GPIO2  (via drill 0.2)
  Top 0.254: v87,74.3 87,73.98 85.57,72.55 66.36,72.55 64.45,74.45 44.13,74.45 42.86,75.72 42.86,97 40.16,99.69 40.16,106.68 39.37,107.47 39.37,111.44 R56.2 | v88.58,72.71 88.27,72.39 88.27,67.94 87,66.67 87,66.52 IC1.51
  Bottom 0.254: v88.58,72.71 v87,74.3
RF_RESETCC  (via drill 0.2, 0.3)
  Top 0.254: IC1.31 86.75,55.09 83.5,58.34 v83.5,64.59 | v54.16,111.58 50.63,111.58 R52.1 | R38.1 v85.91,105.33 v88.66,108.08
  Bottom 0.254: v88.66,108.08 86.91,109.83 55.91,109.83 v54.16,111.58 | v85.91,105.33 85.85,105.27 85.85,102.62 85.34,102.11 85.34,66.43 v83.5,64.59
RF_SFD  (via drill 0.2, 0.3)
  Top 0.254: IC1.42 86.73,60.59 86.36,60.96 v86.36,63.88 | v65.66,109.08 R45.2 | v65.66,109.08
  Bottom 0.254: v65.66,109.08 85.99,109.08 87.38,107.7 87.38,104.14 86.87,103.63 86.87,101.6 86.36,101.09 v86.36,63.88
RF_SIMO  (via drill 0.2, 0.3)
  Top 0.254: IC1.44 93.81,61.59 94.56,62.34 94.56,100.52 90.41,104.66 90.41,111.33 88.66,113.08 v79.16,113.08 | R48.2 66.16,113.58 v65.66,113.08
  Bottom 0.254: v65.66,113.08 v79.16,113.08 88.66,113.08 92.89,108.85 JP5.2
RF_SOMI  (via drill 0.2, 0.3)
  Top 0.254: IC1.43 94.06,61.09 95.06,62.09 95.06,100.78 90.91,104.92 90.91,111.83 88.66,114.08 v79.16,114.08 | R49.2 66.66,115.08 v65.66,114.08
  Bottom 0.254: v65.66,114.08 v79.16,114.08 88.66,114.08 92.16,110.58 94.93,110.58 JP6.2
RF_VREG_EN  (via drill 0.3)
  Top 0.254: IC1.30 86.5,54.59 82.75,58.34 v82.75,63.84 | v84.84,103.63 81.58,103.63 R37.1
  Bottom 0.254: v84.84,103.63 84.84,67.06 83.82,66.04 83.31,66.04 82.8,65.53 82.8,63.89 v82.75,63.84
RX0  (via drill 0.2)
  Top 0.254: v76.52,59.37 77.47,58.42 81.12,58.42 82.5,57.04 IC1.16 | v74.61,59.37 74.61,64.77 73.98,65.41 69.85,65.41 69.69,65.56 v69.69,71.44 | v69.69,73.18 69.53,73.03 66.52,73.03 63.66,75.88 63.66,121.13 SV3.6
  Bottom 0.254: v74.61,59.37 v76.52,59.37 | v69.69,73.18 v69.69,71.44
SCL  (via drill 0.2, 0.3)
  Top 0.254: IC2.6 101.14,61.98 101.08,61.98 101.08,62.24 101.2,62.11 | IC2.6 101.19,59.22 v101.06,59.09 | IC1.38 96.86,58.59 v97.36,58.09 | R32.1 100.41,64.24 101.19,63.45 IC2.6
  Bottom 0.254: v101.06,59.09 | v97.36,58.09 98.36,59.09 v101.06,59.09 | v101.06,59.09
SDA  (via drill 0.2, 0.3)
  Top 0.254: 102.35,61.73 102.6,61.98 102.54,62.04 IC2.5 102.46,60.24 v102.31,60.09 | IC1.39 95.84,59.09 v96.84,60.09
  Top 0.406: IC2.5 102.46,68.68 101.56,69.59 100.47,69.59 R35.1
  Bottom 0.254: v102.31,60.09 | v96.84,60.09 v102.31,60.09 | v102.31,60.09
TCK
  Top 0.254: JTAG.7 45.47,61.97 47.63,61.97 56.52,53.09 IC1.99
TDI
  Top 0.254: JTAG.3 45.55,66.97 47.63,66.97 48.63,65.97 48.63,62.47 57.02,54.09 IC1.97
TDO
  Top 0.254: JTAG.1 45.59,69.47 47.63,69.47 49.13,67.97 49.13,62.72 57.27,54.59 IC1.96
TEST  (via drill 0.3)
  Top 0.254: v49.88,63.97 49.88,62.72 57.52,55.09 IC1.95
  Bottom 0.254: v49.88,63.97 47.46,63.97 JTAG.8
TMS
  Top 0.254: JTAG.5 45.51,64.47 47.63,64.47 48.13,63.97 48.13,62.22 56.77,53.59 IC1.98
TX0  (via drill 0.2, 0.3)
  Top 0.254: v70.96,49.12 69.94,48.1 49.21,48.1 40.8,56.52 40.8,96.36 36.99,100.17 v36.51,100.17 | v35.24,102.08 36.61,103.44 36.61,111.86 42.39,117.63 53.66,117.63 57.15,121.13 SV3.1 | IC1.17 83.03,50.64 83.03,50.01 82.39,49.37 v82.39,48.58 82.39,45.22 76.79,39.62 v76.71,39.62 | v71.12,41.66 v71.12,39.62
  Bottom 0.254: v36.51,100.17 35.88,100.17 35.24,100.81 v35.24,102.08 | v70.96,49.12 71.12,48.96 v71.12,41.66 | v71.12,39.62 v76.71,39.62
V1  (via drill 0.6)
  Top 0.61: v35.05,32 33.96,33.1 L1.1
  Top 0.813: X1.2 4.57,10.92 RF1.1
  Bottom 0.61: R6.2 33.1,14.81 35.05,16.76 v35.05,32
  Bottom 0.813: X1.2 11.72,13.25 13.29,14.81 R6.2
V1+
  Top 0.254: 72.25,47.59 72.5,47.59 75,50.09 IC1.1
  Top 0.406: C27.1 31.25,45.74 33.1,47.59 72.25,47.59
  Top 0.813: R19.2 C25.1 29.25,44.24 30.1,45.09 C27.1
V1-
  Top 0.254: IC1.2 75.5,49.84 72.25,46.59
  Top 0.406: C27.2 32.95,45.69 33.85,46.59 72.25,46.59
  Top 0.813: R20.1 C26.2 33.25,43.94 32.95,44.24 C27.2
V1S
  Top 0.406: X2.2 84.54,19.01 85.34,19.81 OPT1.2
V2
  Top 0.61: L2.1 26.54,28.22 R6.1
  Top 0.813: 18.8,25.1 C2.2 16.72,17.23 X1.1 | 18.8,25.1 L5.1 | 18.8,25.1 29.66,25.1 R6.1
V2S
  Top 0.406: X2.1 79.5,10.2 R62.1
V_CHECK  (via drill 0.2)
  Top 0.254: v86.36,44.32 86.36,41.78 T1.3 | v84.45,58.29 84.45,64.14 84.91,64.59 IC1.50
  Bottom 0.254: v86.36,44.32 87.63,44.32 88.9,45.59 88.9,50.67 88.27,51.31 88.27,52.58 90.81,55.12 90.81,55.75 90.17,56.39 86.36,56.39 v84.45,58.29
VASYS
  Top 0.254: 79.5,49.06 IC1.10 | 79.5,49.06 C13.1 | 79.5,49.06 81.09,49.06 C11.2
VCORE
  Top 0.254: IC1.23 86,49.59 | IC1.23 | 86,49.59 | C14.2 87.15,48.44 86,49.59
VDSYS
  Top 0.254: IC1.20 84.5,49.21 84.25,48.96 C9.2 84.9,48.31 85.56,47.65 C6.2
  Top 0.305: C18.2 72.75,66.86 72.75,67.34 73,67.59 75.25,67.59 75.5,67.34 IC1.74 75.5,64.74 77.22,63.03 77.22,59.44 77.72,58.93 81.28,58.93 85.85,54.36 | C16.2 IC1.26 87.62,52.59 85.85,54.36 | C16.2 | IC1.20 84.5,53 85.85,54.36
VREF
  Top 0.254: IC1.7 78,48.59 77.5,48.09 C7.1 | C7.1
XIN1
  Top 0.254: IC1.24 86.49,50.38 86.49,49.85 86.75,49.59 90.06,49.59 Q1.2
XOUT1
  Top 0.254: IC1.25 89.7,50.79 90,51.09 91.5,51.09 91.75,50.84 91.75,50.07 Q1.1

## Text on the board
tPlace: Level 1&2 EVSE | GND | +5V | GND | GND | External / VIN | -12V | +12V | +3V3 | TIDA-00637 | PSU | EXT | R4 | R3 | R2 | R1 | +V | Relay / Outputs | L1 | L2 | C1 | C2 | PILOT | GFCI / IN | GFCI / TEST | RELAY / CHECK
bNames: + | +
_tplace: R49 | SV1 | R53 | SV2 | R48 | DVCC | SV3 | DGND | R47 | R46 | C39 | R56 | R52 | C42 | R45 | C40 | R55 | R44 | R40 | R36 | R51 | R43 | C41 | R39 | R42 | R38 | JP5 | JP6 | RF2 | RF1 | R37 | OK2 | R54 | RS1 | IRDA | 1 | 1 | JP8 | R50 | REACT | OK1 | JP7 | 5 | 9 | 4 | R41 | 8 | 3 | ACT | 7 | 2 | 6 | LED2 | 1 | R5 | R4 | LCD1 | LED1 | R35 | JP1 | C37 | DVCC | R32 | 1 | INTERNAL | MSP430F673x 1-Phase Energy Meter | C18 | Version 2.4 | EXTERNAL | JP4 | DVCC | VCC_PL | IC1 | S1 | IC2 | VCC_EXT | R31 | R30 | R1 | RTH | R3 | C15 | C17 | RESET | C16 | C6 | R27 | C7 | C31 | R24 | C27 | C13 | C11 | C9 | C14 | R28 | R25 | Q1 | C30 | C25 | C26 | C19 | C23 | C21 | C24 | C2 | C4 | R26 | R29 | C1 | C3 | U1 | R19 | R20 | R12 | C20 | R14 | C22 | JTAG | * | C35 | R18 | R17 | R9 | R13 | R10 | R15 | D13 | R23 | R11 | R16 | R7 | R8 | C32 | D11 | D12 | JP2 | C33 | C34 | AUX1 | AUX2 | AUX3 | L3 | L4 | L5 | L6 | R21 | D9 | D10 | JP3 | GND | C28 | R34 | VCC_EXT | D2 | D4 | D6 | D8 | C38 | D1 | D3 | D5 | D7 | S3 | R22 | R6 | R33 | L1 | L2 | 120mA MAX | S2 | C36 | LINE | NEUTRAL | 120/240 Vrms | Warning: | CUR1+ | CUR1- | CUR2+ | CUR2- | 60/50 Hz | 3VA | High Voltage
_bplace: D15 | + | C44 | R62 | D16 | C45 | + | U2 | D17 | C43 | D14 | R58 | R59 | T1 | R61 | R65 | R60 | R66 | T2 | R64 | R63 | R57 | U3 | R2 | C8 | C10 | C29 | C5 | C12 | L7 | ELLCTV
